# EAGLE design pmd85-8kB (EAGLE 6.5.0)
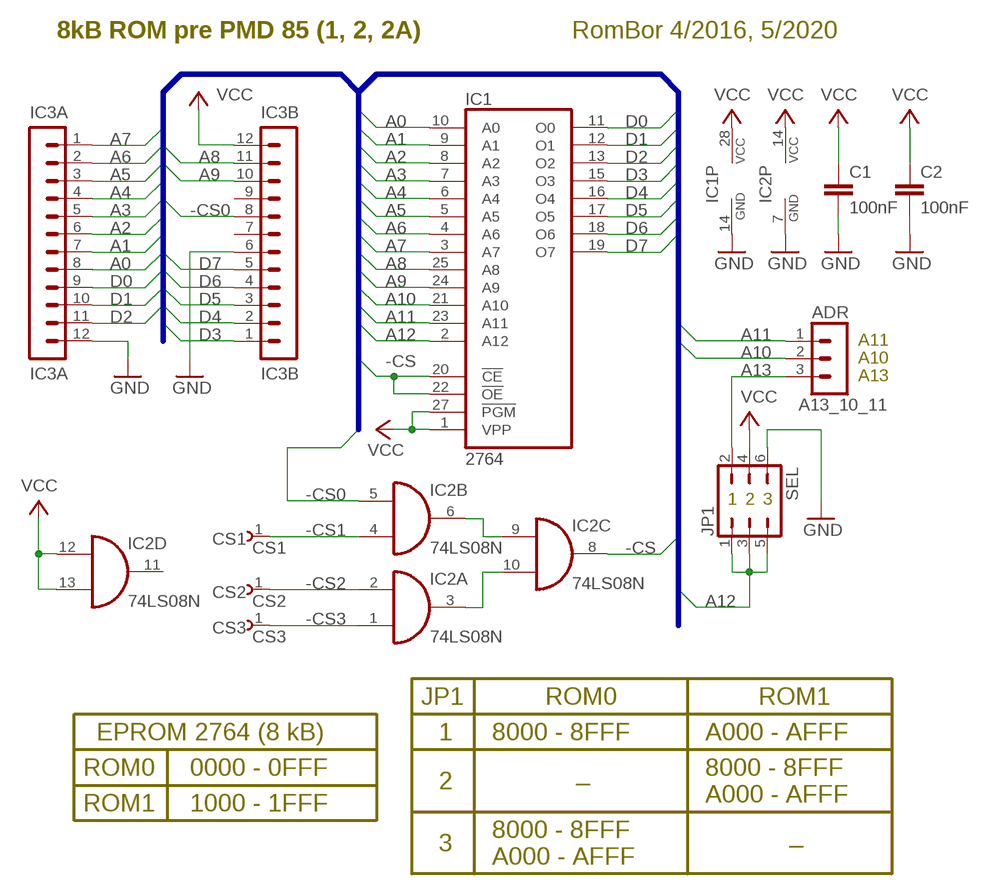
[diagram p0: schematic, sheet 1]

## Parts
A13_10_11  ADR  MA03-1  [MA03-1]
C1  100nF  C2.5/2  [C2.5-2]
C2  100nF  C2.5/2  [C2.5-2]
CS1  CS1  PINHD-1X1  [1X01]
CS2  CS2  PINHD-1X1  [1X01]
CS3  CS3  PINHD-1X1  [1X01]
IC1  2764  [DIL28]
IC2  74LS08N  [DIL14]
IC3A  IC3A  MA12-1  [MA12-1]
IC3B  IC3B  MA12-1  [MA12-1]
JP1  SEL  JP3Q  [JP3Q]

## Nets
-CS: IC1.20(!CE) IC1.22(!OE) IC2.8(C:O)
-CS0: IC2.5(B:I1) IC3B.8
-CS1: CS1.1 IC2.4(B:I0)
-CS2: CS2.1 IC2.2(A:I1)
-CS3: CS3.1 IC2.1(A:I0)
A0: IC1.10(A0) IC3A.8
A1: IC1.9(A1) IC3A.7
A2: IC1.8(A2) IC3A.6
A3: IC1.7(A3) IC3A.5
A4: IC1.6(A4) IC3A.4
A5: IC1.5(A5) IC3A.3
A6: IC1.4(A6) IC3A.2
A7: IC1.3(A7) IC3A.1
A8: IC1.25(A8) IC3B.11
A9: IC1.24(A9) IC3B.10
A10: A13_10_11.2 IC1.21(A10)
A11: A13_10_11.1 IC1.23(A11)
A12: IC1.2(A12) JP1.1 JP1.3 JP1.5
A13: A13_10_11.3 JP1.2
D0: IC1.11(O0) IC3A.9
D1: IC1.12(O1) IC3A.10
D2: IC1.13(O2) IC3A.11
D3: IC1.15(O3) IC3B.1
D4: IC1.16(O4) IC3B.2
D5: IC1.17(O5) IC3B.3
D6: IC1.18(O6) IC3B.4
D7: IC1.19(O7) IC3B.5
GND: C1.2 C2.2 IC1.14(GND) IC2.7(P:GND) IC3A.12 IC3B.6 JP1.6
N$1: IC2.3(A:O) IC2.10(C:I1)
N$2: IC2.6(B:O) IC2.9(C:I0)
VCC: C1.1 C2.1 IC1.1(VPP) IC1.27(!PGM) IC1.28(VCC) IC2.12(D:I0) IC2.13(D:I1) IC2.14(P:VCC) IC3B.12 JP1.4
Unconnected: IC2.11(D:O) IC3B.7 IC3B.9

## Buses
A[0..12],D[0..7],-CS0,-CS

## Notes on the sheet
- 8kB ROM pre PMD 85 (1, 2, 2A) | RomBor 4/2016, 5/2020
- A11
- A10
- A13
- 1 | 2 | 3
- JP1 | ROM0 | ROM1
- EPROM 2764 (8 kB) | 1 | 8000 - 8FFF | A000 - AFFF
- ROM0 | 0000 - 0FFF | _ | 8000 - 8FFF
- 2
- A000 - AFFF
- ROM1 | 1000 - 1FFF
- 8000 - 8FFF | _
- 3
- A000 - AFFF

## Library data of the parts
A13_10_11 = con-lstb:MA03-1: PIN HEADER; OC_FARNELL: unknown; OC_NEWARK: unknown
C1 C2 = capacitor-wima:C: CAPACITOR
CS1-CS3 = pinhead_MP_08mm:PINHD-1X1: PIN HEADER
IC1 = memory:2764: MEMORY
IC2 = 74xx-eu:74*08: Quad 2-input AND gate
IC3A IC3B = con-lstb:MA12-1: PIN HEADER; OC_FARNELL: unknown; OC_NEWARK: unknown
JP1 = jumper:JP3Q: JUMPER

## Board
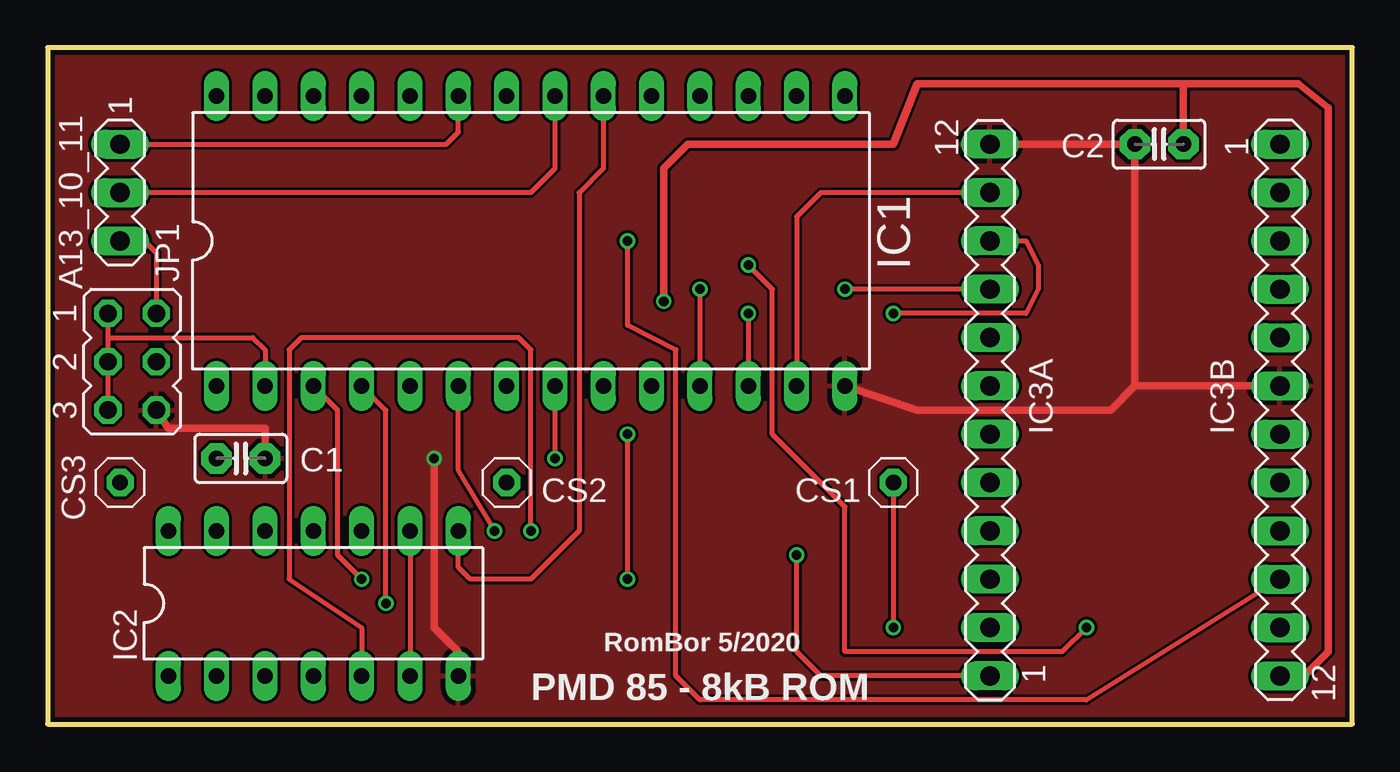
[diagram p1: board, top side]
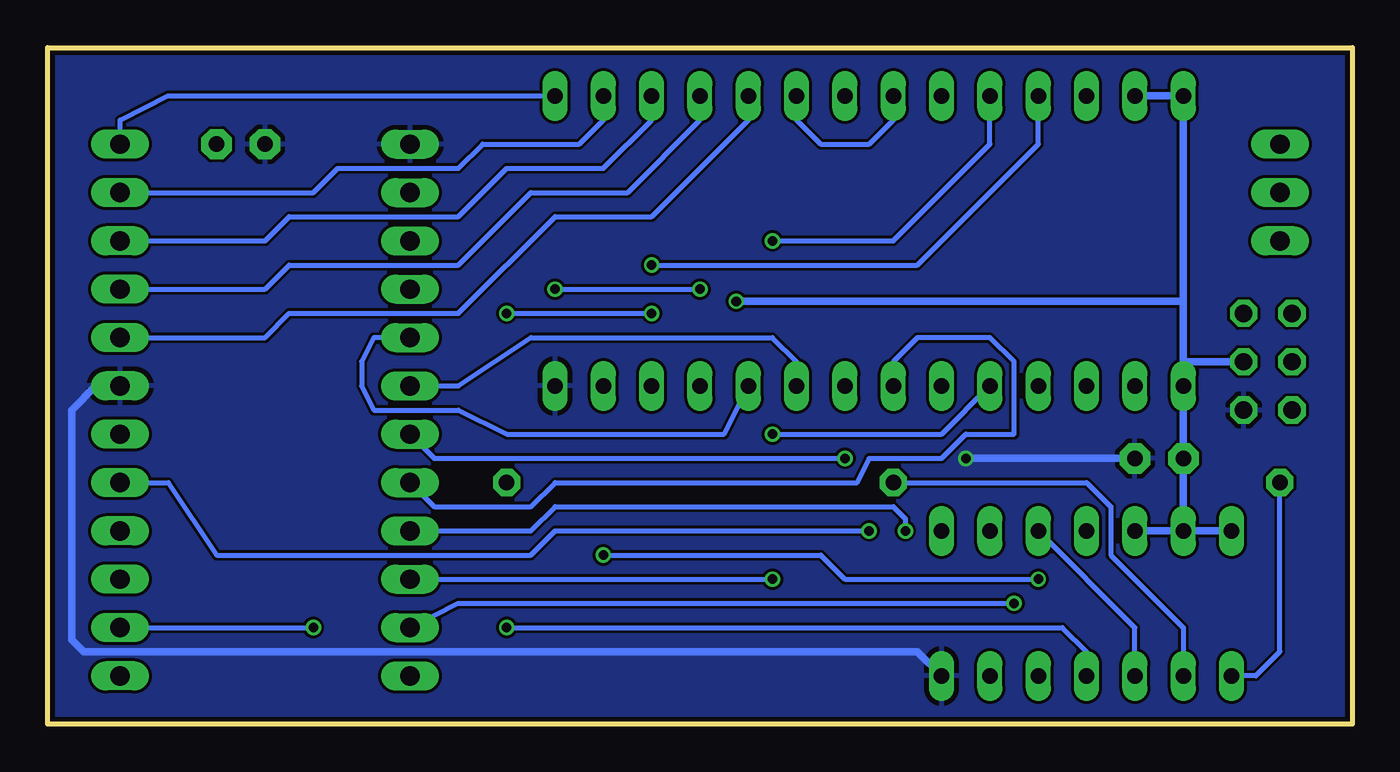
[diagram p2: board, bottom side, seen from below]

Size 68.58 x 35.56 mm. Coordinates in mm from the lower left corner, seen from the top.
Outline: 0,0 68.58,0 68.58,35.56 0,35.56 0,0
Copper layers (1*16): Top 0.035mm / dielectric 1.5mm / Bottom 0.035mm
Design rules "SeeedStudio_2layer_DRU_no_angle_20140221": minimum track width 6mil, minimum drill 12mil, track to track 6mil, track to pad 6mil, pad to pad 6mil, via to via 6mil, smd to smd 0mil, copper to edge 10mil, drill to drill 10mil, minimum pad ring 10mil, minimum via ring 6mil, stop-mask expansion 2mil, vias tented up to drill 100mil, thermal gap 10mil

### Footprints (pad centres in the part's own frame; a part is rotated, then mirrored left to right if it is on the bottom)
MA03-1 = drill 1.016 long: 1 -2.54,0; 2 0,0; 3 2.54,0
C2.5-2 = drill 0.813 pad 1.6 octagon: 1 -1.27,0; 2 1.27,0
1X01 = drill 0.813 pad 1.422 octagon: 1 0,0
DIL28 = drill 0.813 long: 1 -16.51,-7.62; 2 -13.97,-7.62; 3 -11.43,-7.62; 4 -8.89,-7.62; 5 -6.35,-7.62; 6 -3.81,-7.62; 7 -1.27,-7.62; 8 1.27,-7.62; 9 3.81,-7.62; 10 6.35,-7.62; 11 8.89,-7.62; 12 11.43,-7.62; 13 13.97,-7.62; 14 16.51,-7.62; 15 16.51,7.62; 16 13.97,7.62; 17 11.43,7.62; 18 8.89,7.62; 19 6.35,7.62; 20 3.81,7.62; 21 1.27,7.62; 22 -1.27,7.62; 23 -3.81,7.62; 24 -6.35,7.62; 25 -8.89,7.62; 26 -11.43,7.62; 27 -13.97,7.62; 28 -16.51,7.62
DIL14 = drill 0.813 long: 1 -7.62,-3.81; 2 -5.08,-3.81; 3 -2.54,-3.81; 4 0,-3.81; 5 2.54,-3.81; 6 5.08,-3.81; 7 7.62,-3.81; 8 7.62,3.81; 9 5.08,3.81; 10 2.54,3.81; 11 0,3.81; 12 -2.54,3.81; 13 -5.08,3.81; 14 -7.62,3.81
MA12-1 = drill 1.016 long: 1 -13.97,0; 2 -11.43,0; 3 -8.89,0; 4 -6.35,0; 5 -3.81,0; 6 -1.27,0; 7 1.27,0; 8 3.81,0; 9 6.35,0; 10 8.89,0; 11 11.43,0; 12 13.97,0
JP3Q = drill 0.914 octagon: 1 -2.54,-1.27; 2 -2.54,1.27; 3 0,-1.27; 4 0,1.27; 5 2.54,-1.27; 6 2.54,1.27

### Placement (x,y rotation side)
A13_10_11  3.81,27.94 270 top
C1  10.16,13.97 0 top
C2  58.42,30.48 180 top
CS1  44.45,12.7 0 top
CS2  24.13,12.7 0 top
CS3  3.81,12.7 0 top
IC1  25.4,25.4 0 top
IC2  13.97,6.35 0 top
IC3A  49.53,16.51 90 top
IC3B  64.77,16.51 270 top
JP1  4.45,19.05 270 top

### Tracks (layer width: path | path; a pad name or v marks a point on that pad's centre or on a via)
-CS
  Top 0.254: IC1.20 29.21,29.21 27.94,27.94 27.94,10.16 25.4,7.62 22.23,7.62 21.59,8.26 IC2.8
  Bottom 0.254: IC1.22 24.13,31.75 25.4,30.48 27.94,30.48 29.21,31.75 IC1.20
-CS0  (via drill 0.5)
  Top 0.254: v25.4,10.16 25.4,19.68 24.77,20.32 13.34,20.32 12.7,19.68 12.7,7.62 16.51,5.08 IC2.5
  Bottom 0.254: v25.4,10.16 41.91,10.16 43.18,8.89 59.69,8.89 62.23,12.7 IC3B.8
-CS1  (via drill 0.5)
  Top 0.254: CS1.1 v44.45,5.08
  Bottom 0.254: v44.45,5.08 15.24,5.08 13.97,3.81 IC2.4
-CS2
  Bottom 0.254: CS2.1 13.97,12.7 12.7,11.43 12.7,8.89 8.89,5.08 IC2.2
-CS3
  Bottom 0.254: CS3.1 3.81,3.81 5.08,2.54 IC2.1
A0
  Bottom 0.254: IC1.10 33.02,15.24 44.45,15.24 46.99,16.51 51.44,16.51 52.07,17.78 52.07,19.05 51.44,20.32 IC3A.8
A1
  Bottom 0.254: IC1.9 29.21,19.05 30.48,20.32 43.18,20.32 46.99,17.78 IC3A.7
A2  (via drill 0.5)
  Top 0.254: v26.67,13.97 IC1.8
  Bottom 0.254: v26.67,13.97 48.26,13.97 IC3A.6
A3
  Bottom 0.254: IC1.7 24.13,19.05 22.86,20.32 19.05,20.32 17.78,19.05 17.78,15.24 20.32,15.24 21.59,13.97 25.4,13.97 26.04,12.7 41.91,12.7 43.18,11.43 48.26,11.43 IC3A.5
A4  (via drill 0.5)
  Top 0.254: v23.5,10.16 21.59,13.34 IC1.6
  Bottom 0.254: v23.5,10.16 23.5,10.79 24.13,11.43 41.91,11.43 43.18,10.16 IC3A.4
A5  (via drill 0.5)
  Top 0.254: v30.48,7.62 v30.48,15.24
  Bottom 0.254: IC1.5 21.59,15.24 v30.48,15.24 | IC3A.3 v30.48,7.62
A6  (via drill 0.5)
  Top 0.254: IC1.4 17.78,16.51 v17.78,6.35
  Bottom 0.254: v17.78,6.35 46.99,6.35 IC3A.2
A7  (via drill 0.5)
  Top 0.254: IC1.3 15.24,16.51 15.24,8.89 v16.51,7.62 | v39.37,8.89 39.37,3.81 40.64,2.54 IC3A.1
  Bottom 0.254: v16.51,7.62 26.67,7.62 27.94,8.89 v39.37,8.89
A8  (via drill 0.5, 0.5 pad 0.41)
  Top 0.254: v36.83,24.13 38.1,22.86 38.1,15.24 41.91,11.43 41.91,3.81 53.34,3.81 v54.61,5.08
  Bottom 0.254: IC1.25 16.51,30.48 22.86,24.13 v36.83,24.13 | IC3B.11 v54.61,5.08
A9  (via drill 0.5 pad 0.41)
  Top 0.254: v30.48,25.4 30.48,20.95 33.02,19.68 33.02,2.54 34.29,1.27 54.61,1.27 IC3B.10
  Bottom 0.254: IC1.24 19.05,30.48 24.13,25.4 v30.48,25.4
A10
  Top 0.254: IC1.21 26.67,29.21 25.4,27.94 A13_10_11.2
A11
  Top 0.254: A13_10_11.1 20.95,30.48 21.59,31.11 IC1.23
A12
  Top 0.254: JP1.5 JP1.3 3.17,20.32 | IC1.2 11.43,19.68 10.79,20.32 3.17,20.32 | JP1.1 3.17,20.32
A13
  Top 0.254: A13_10_11.3 5.08,25.4 5.71,24.77 JP1.2
D0  (via drill 0.5, 0.5 pad 0.41)
  Top 0.254: v34.29,22.86 IC1.11 | IC3A.9 v41.91,22.86
  Bottom 0.254: v41.91,22.86 v34.29,22.86
D1  (via drill 0.5, 0.5 pad 0.41)
  Top 0.254: v36.83,21.59 IC1.12 | v44.45,21.59 51.44,21.59 52.07,22.86 52.07,24.13 51.44,25.4 IC3A.10
  Bottom 0.254: v44.45,21.59 v36.83,21.59
D2
  Top 0.254: IC1.13 39.37,26.67 40.64,27.94 IC3A.11
D3
  Bottom 0.254: IC3B.1 64.77,31.75 62.23,33.02 IC1.15
D4
  Bottom 0.254: IC3B.2 54.61,27.94 53.34,29.21 46.99,29.21 45.72,30.48 40.64,30.48 39.37,31.75 IC1.16
D5
  Bottom 0.254: IC3B.3 57.15,25.4 55.88,26.67 46.99,26.67 44.45,29.21 39.37,29.21 36.83,31.75 IC1.17
D6
  Bottom 0.254: IC3B.4 57.15,22.86 55.88,24.13 46.99,24.13 43.18,27.94 38.1,27.94 34.29,31.75 IC1.18
D7
  Bottom 0.254: IC3B.5 57.15,20.32 55.88,21.59 46.99,21.59 41.91,26.67 36.83,26.67 31.75,31.75 IC1.19
GND  (via drill 0.5)
  Top 0.406: IC3B.6 57.15,17.78 | 57.15,17.78 C2.2 IC3A.12 | IC1.14 45.72,16.51 55.88,16.51 57.15,17.78 | v20.32,13.97 20.32,5.08 21.59,3.81 IC2.7 | JP1.6 6.35,15.56 11.43,15.56 C1.2
  Bottom 0.406: C1.2 v20.32,13.97 | IC3B.6 66.04,17.78 67.31,16.51 67.31,4.45 66.67,3.81 22.86,3.81 IC2.7
  pour Top: 0,35.56 68.58,35.56 68.58,0 0,0
  pour Bottom: 0,35.56 68.58,35.56 68.58,0 0,0
N$1
  Bottom 0.254: IC2.3 11.43,5.08 IC2.10
N$2
  Top 0.254: IC2.9 IC2.6
VCC  (via drill 0.5)
  Top 0.406: IC3B.12 66.04,2.54 67.31,3.81 67.31,32.38 65.72,33.66 59.69,33.66 | 59.69,33.66 45.72,33.66 44.45,30.48 33.66,30.48 32.38,29.21 v32.38,22.23 | C2.1 59.69,33.66
  Bottom 0.406: 8.89,19.05 IC1.1 C1.1 IC2.13 | 8.89,19.05 8.89,22.23 | 8.89,22.23 IC1.28 IC1.27 | 8.89,22.23 v32.38,22.23 | 8.89,19.05 JP1.4 | IC2.12 IC2.13 | IC2.14 IC2.13

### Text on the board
tPlace: RomBor 5/2020 | PMD 85 - 8kB ROM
